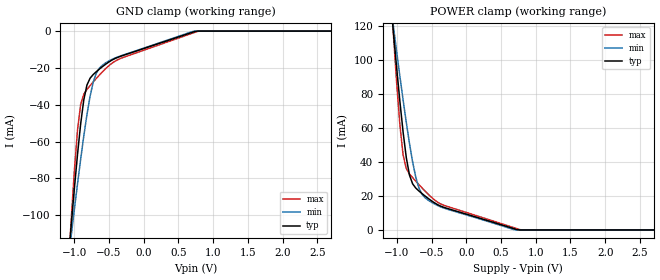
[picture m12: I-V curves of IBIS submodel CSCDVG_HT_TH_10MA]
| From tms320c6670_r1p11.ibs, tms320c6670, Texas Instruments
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|   Model Cell CSCDVG_HT_TH_10MA
|CSCDVG_HT_TH_10MA
[Submodel]   CSCDVG_HT_TH_10MA
Submodel_type   Dynamic_clamp
[POWER_clamp]
|   voltage   I(typ)   I(min)   I(max)
-1.5V     334.6mA    270.5mA    430.2mA
-1.091V   135.2mA    133mA      142mA
-1.046V   114.4mA    118.4mA    112.7mA
-954.6mV  74.94mA    89.89mA    61.12mA
-909.2mV  57.31mA    76.22mA    43.91mA
-818.2mV  32.28mA    50.96mA    32.96mA
-727.3mV  24.63mA    31.02mA    28.68mA
-636.4mV  21.35mA    20.92mA    24.66mA
-545.5mV  18.44mA    17.41mA    20.87mA
-318.2mV  13.23mA    12.8mA     14.44mA
772.8mV   0A         0A         196.8uA
3V        0A         0A         0A
[GND_clamp]
|   voltage   I(typ)   I(min)   I(max)
-1.5V     -325.3mA   -263mA     -419.1mA
-1.091V   -126.2mA   -125.8mA   -131.6mA
-1.046V   -105.6mA   -111.2mA   -102.8mA
-954.6mV  -67.09mA   -83.04mA   -53.93mA
-909.2mV  -50.45mA   -69.63mA   -39.86mA
-863.7mV  -37.29mA   -56.94mA   -34.26mA
-818.2mV  -29.27mA   -45.31mA   -31.67mA
-727.3mV  -23.55mA   -27.6mA    -27.59mA
-636.4mV  -20.53mA   -19.98mA   -23.76mA
-545.5mV  -17.88mA   -17.17mA   -20.27mA
772.8mV   0A         0A         -190.4uA
3V        0A         0A         0A
